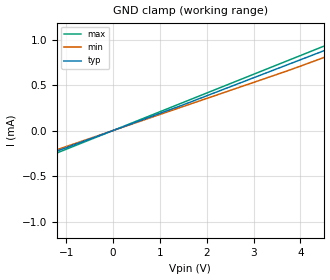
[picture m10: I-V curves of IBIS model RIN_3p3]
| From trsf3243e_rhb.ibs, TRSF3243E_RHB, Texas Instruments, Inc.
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[Model]   RIN_3p3
Model_type   Input
Vinl = 0.6
Vinh = 2.4
|   typ   min   max
C_comp   1.07pF   0.83pF   1.45pF
[Voltage Range]   3.3   3   3.6
[Temperature Range]   27   110   -40
[Power Clamp Reference]   3.3   3   3.6
[GND Clamp Reference]   0   0   0
[GND Clamp]
|   Voltage   I(typ)   I(min)   I(max)
-25V      -5.173mA   -4.828mA   -5.656mA
-11.85V   -2.436mA   -2.273mA   -2.665mA
-3.868V   -776.6uA   -723.4uA   -850.7uA
-1.208V   -227.4uA   -212.4uA   -248.6uA
1.517V    286.1uA    267.5uA    312.5uA
3.607V    699.5uA    635.3uA    742.5uA
5.473V    1.069mA    989.2uA    1.138mA
6.03V     1.179mA    1.096mA    1.264mA
6.27V     1.226mA    1.143mA    1.318mA
25V       5.106mA    4.777mA    5.57mA
